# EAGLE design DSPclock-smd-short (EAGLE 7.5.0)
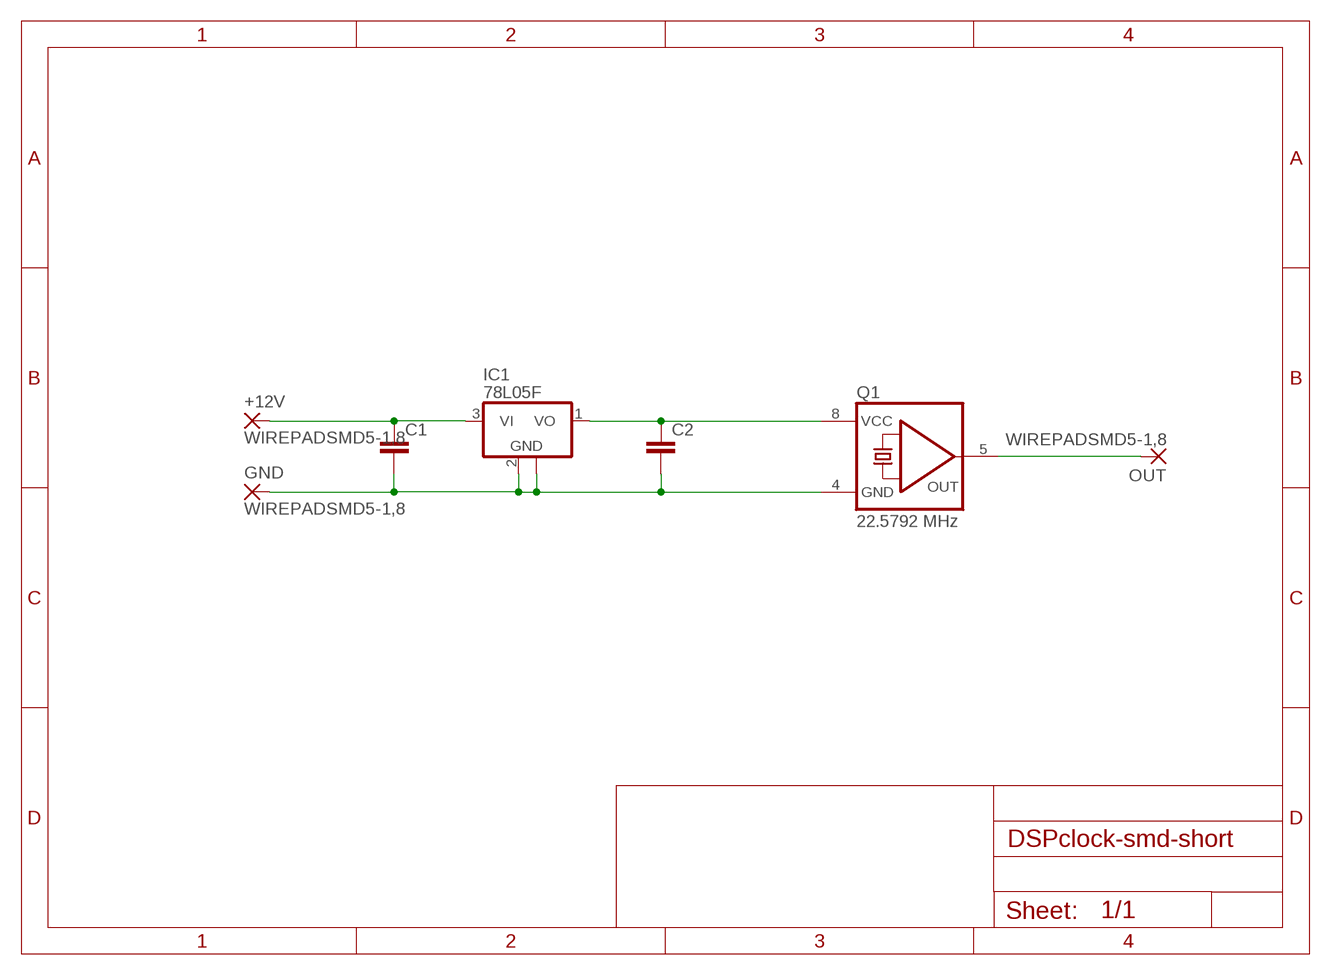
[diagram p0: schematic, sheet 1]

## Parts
+12V  WIREPADSMD5-1,8  [5-1,8]
C1  C-EUC1206  [C1206]
C2  C-EUC1206  [C1206]
GND  WIREPADSMD5-1,8  [5-1,8]
IC1  78L05F  [SOT89]
OUT  WIREPADSMD5-1,8  [5-1,8]
Q1  22.5792 MHz  QG5460  [DIL08S]

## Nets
5V: C2.1 IC1.1(VO) Q1.8(VCC)
12V: +12V.1(P) C1.1 IC1.3(VI)
FOUT: OUT.1(P) Q1.5(OUT)
GND: C1.2 C2.2 GND.1(P) IC1.2(GND) IC1.2@1(GND) Q1.4(GND)

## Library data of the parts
+12V GND OUT = wirepad:WIREPAD: Wire PAD connect wire on PCB
C1 C2 = rcl:C-EU: CAPACITOR, European symbol
IC1 = linear:78L*: POSITOIV-VOLTAGE REGULATORS Output up to 100 mA Source: Datasheet
Q1 = crystal:QG5460: CRYSTAL RESONATOR; OC_FARNELL: unknown; OC_NEWARK: unknown

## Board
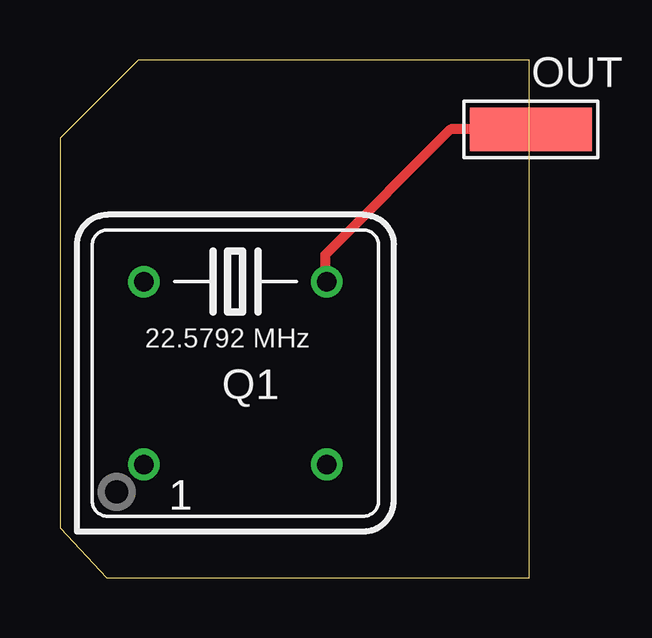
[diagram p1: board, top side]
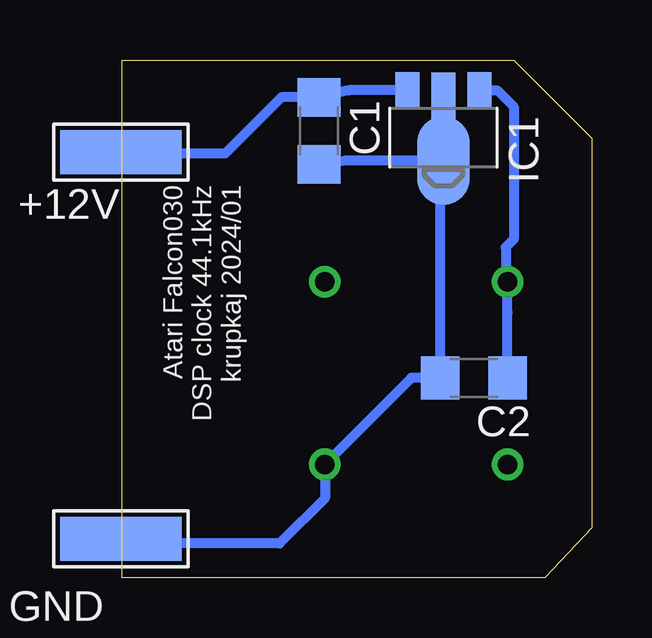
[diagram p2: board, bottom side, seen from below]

Size 19.57 x 21.59 mm. Coordinates in mm from the lower left corner, seen from the top.
Outline: 19.57,0 19.57,21.59 3.25,21.59 0,18.34 0,2.08 1.95,0 19.57,0
Copper layers (1*16): Top 0.035mm / dielectric 1.5mm / Bottom 0.035mm
Design rules "default": minimum track width 10mil, minimum drill 24mil, track to track 8mil, track to pad 8mil, pad to pad 8mil, via to via 8mil, smd to smd 8mil, copper to edge 40mil, drill to drill 8mil, minimum pad ring 10mil, minimum via ring 8mil, stop-mask expansion 4mil, vias tented up to drill 0mil, thermal gap 10mil

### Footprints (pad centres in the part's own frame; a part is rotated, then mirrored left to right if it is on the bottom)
5-1,8 = smd 1.829 x 5.08: 1 0,0
C1206 = smd 1.6 x 1.8: 1 -1.4,0; 2 1.4,0
SOT89 = smd 1 x 1.5: 1 -1.499,-1.981; 3 1.499,-1.981 | smd 1 x 2: 2 0,-1.727 | smd 2.2 x 3.7: 2@1 0,0.94
DIL08S = drill 0.813: 1 -3.81,-3.81; 4 3.81,-3.81; 5 3.81,3.81; 8 -3.81,3.81

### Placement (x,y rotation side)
+12V  19.63,17.74 90 bottom
C1  11.37,18.63 270 bottom
C2  4.91,8.33 180 bottom
GND  19.63,1.63 90 bottom
IC1  6.18,18.34 180 bottom
OUT  19.63,18.69 90 top
Q1  7.32,8.53 0 top

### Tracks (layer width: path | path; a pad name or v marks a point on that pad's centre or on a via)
5V
  Bottom 0.406: C2.1 3.51,11.04 Q1.8 3.58,12.41 3.58,13.79 3.25,14.11 3.25,19.64 3.93,20.32 IC1.1
12V
  Bottom 0.406: IC1.3 10.11,20.32 C1.1 12.94,20.03 15.28,17.69 19.58,17.69 +12V.1
FOUT
  Top 0.406: OUT.1 16.29,18.69 11.05,13.46 11.05,12.41 Q1.5
GND
  Bottom 0.406: IC1.2 IC1.2@1 | GND.1 19.43,1.43 13.01,1.43 11.13,3.31 Q1.4 7.52,8.33 C2.2 6.31,16.94 IC1.2@1 | IC1.2@1 10.23,17.4 C1.2

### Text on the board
bNames: Atari Falcon030 / DSP clock 44.1kHz / krupkaj 2024/01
